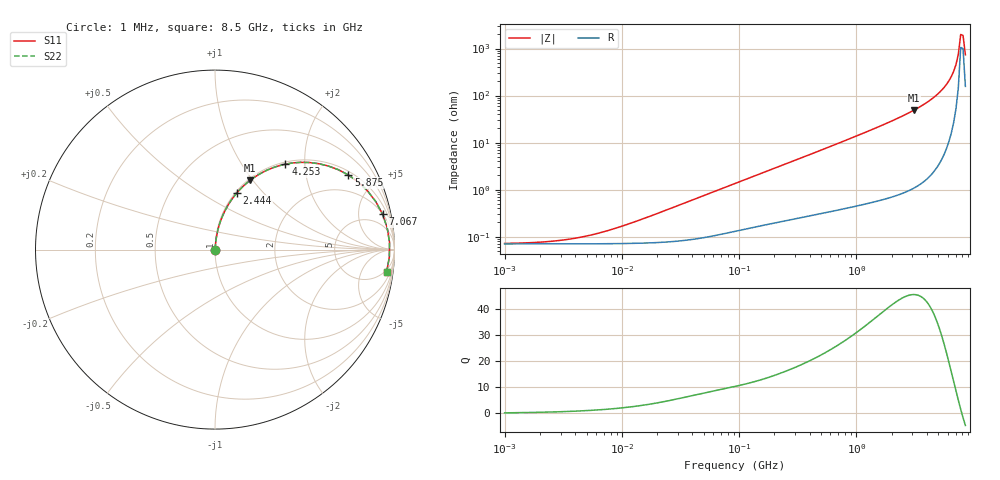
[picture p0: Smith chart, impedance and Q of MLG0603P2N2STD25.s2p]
! S-Parameter Data Generated by TDK Corporation
! Copyright(C) 2025 TDK Corporation.
! All Rights Reserved.
! TDK P/N: MLG0603P2N2STD25 (SMD / SMT Inductor (Coil))
! Property: L=2.2nH at 500MHz
! Size(LxWxT): 0.6x0.3x0.3mm
! Model Type: s2p (Touchstone File Format Version 1.0)
! Frequency: DC=Yes Start=1MHz Stop=8500MHz 198points Log-sweep
! Model Generated on Feb. 6, 2025
! Terms and conditions regarding TDK Simulation Models:
! 1)This simulation model is being provided solely for informational
!  purposes. Please refer to the specifications of the products in
!  terms of detailed characteristics of such products.
! 2)In no event shall TDK Corporation of any of its subsidiaries be
!  liable for any loss or damage arising, directly or indirectly,
!  from any information contained in this simulation model, including,
!  but not limited to loss or damages arising from any inaccuracies,
!  omissions or errors in connection with such information.
! 3)Any and all copyrights on this simulation model are owned by
!  TDK Corporation.  Duplication or redistribution of this simulation
!  model without prior written permission from TDK Corporation
!  is prohibited.
! 4)This simulation model is subject to any modification or change
!  without any prior notice.
! 5)Neither TDK Corporation nor any of its subsidiaries shall make any
!  warranty, express or implied, including but not limited to the
!  correctness, implied warranties of merchantability and fitness for
!  a particular purpose with respect to this simulation models.
! 6)The use of this simulation model shall be deemed to have consented
!  to the terms and conditions hereof.
! Port Assignments:
!  1 ---@@@--- 2
! Applicable Conditions:
!  Temperature = 25 degC
!  DC Bias Current = 0 A
!  Small Signal Operation
# Hz S MA R 50
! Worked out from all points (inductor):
!   197 points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, 1 MHz to 8.5 GHz, reference 50 ohm
!   read as one part in series: L = 2.4 nH near 14.55 MHz
!   highest Q = 45.4 at 3.079 GHz (marker M1), where L = 2.51 nH
!   self-resonance near 7.75 GHz
!   S11 on the Smith chart (normalised r, x): 1 MHz: 1.00, +0.00; 2.444 GHz: 1.02, +0.73; 4.253 GHz: 1.04, +1.60; 5.875 GHz: 1.15, +3.48; 7.067 GHz: 2.06, +9.08; 8.5 GHz: 4, -14
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1000000  0.0007157 12.2  0.9993 -0.0  0.9993 -0.0  0.0007157 12.2
2403882  0.0007885 27.3  0.9993 -0.0  0.9993 -0.0  0.0007885 27.3
4587603  0.0009855 44.5  0.9993 -0.0  0.9993 -0.0  0.0009855 44.5
8755050  0.001498 61.7  0.9993 -0.1  0.9993 -0.1  0.001498 61.7
2.10461e7  0.00325 76.4  0.9992 -0.2  0.9992 -0.2  0.00325 76.4
9.219544e7  0.01345 83.7  0.9986 -0.8  0.9986 -0.8  0.01345 83.7
4.229561e8  0.05843 83.9  0.9955 -3.3  0.9955 -3.3  0.05843 83.9
9.708683e8  0.1323 80.5  0.9869 -7.6  0.9869 -7.6  0.1323 80.5
1.940355e9  0.2663 73.2  0.9574 -15.4  0.9574 -15.4  0.2663 73.2
2.444114e9  0.3389 68.9  0.9332 -19.8  0.9332 -19.8  0.3389 68.9
3.07866e9  0.4337 63.0  0.8916 -25.7  0.8916 -25.7  0.4337 63.0
3.703002e9  0.5305 56.7  0.8358 -32.0  0.8358 -32.0  0.5305 56.7
4.253027e9  0.6171 50.5  0.7719 -38.1  0.7719 -38.1  0.6171 50.5
5.115526e9  0.7494 39.7  0.6393 -48.5  0.6393 -48.5  0.7494 39.7
5.87536e9  0.8514 29.2  0.4889 -58.3  0.4889 -58.3  0.8514 29.2
6.44363e9  0.9109 21.0  0.3595 -65.4  0.3595 -65.4  0.9109 21.0
6.748056e9  0.9351 16.6  0.2864 -68.7  0.2864 -68.7  0.9351 16.6
7.066863e9  0.9541 12.0  0.2087 -71.4  0.2087 -71.4  0.9541 12.0
7.400733e9  0.9671 7.2  0.128 -71.5  0.128 -71.5  0.9671 7.2
7.750377e9  0.9733 2.4  0.04878 -55.6  0.04878 -55.6  0.9733 2.4
8.116539e9  0.9723 -2.5  0.05106 55.9  0.05106 55.9  0.9723 -2.5
8.5e9  0.9642 -7.3  0.1303 70.4  0.1303 70.4  0.9642 -7.3
